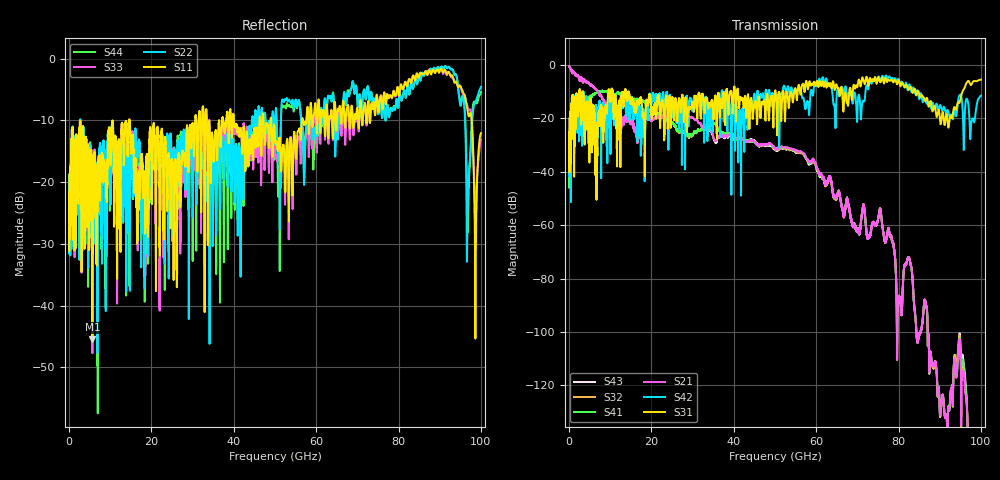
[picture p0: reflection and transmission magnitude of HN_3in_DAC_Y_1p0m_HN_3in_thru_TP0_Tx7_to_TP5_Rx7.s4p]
# GHz S RI R 45
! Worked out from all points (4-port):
!   4000 points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, 25 MHz to 100 GHz, reference 45 ohm
!   strongest paths, dB at 25 MHz, 25.02 GHz, 50.02 GHz, 75.03 GHz, 100 GHz:
!     S31: -39.1, -12.4, -9.7, -4.6, -5.5
!     S42: -38.9, -15.9, -12.9, -4.7, -11.5
!     S21: -0.4, -19.1, -31.1, -57.7, -180.1
!     S41: -45.9, -21.3, -31.3, -57.7, -182.6
!     S32: -45.9, -21.5, -31.2, -57.7, -181.7
!     S43: -0.4, -19.2, -31.5, -57.7, -174.4
!   lowest |S11| = -45.4 dB at 5.675 GHz (marker M1), VSWR 1.01, Z = 44.9 + j0.463 ohm
!   |S11| at or under -10 dB: start of sweep to 10.55 GHz; 14.73 GHz to 30.62 GHz (15.89 GHz wide, 70.1 % of centre); 49.09 GHz to 56.56 GHz (7.47 GHz wide, 14.1 % of centre)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
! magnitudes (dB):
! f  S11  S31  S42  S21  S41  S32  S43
! 25 MHz  -24.2  -39.1  -38.9  -0.4  -45.9  -45.9  -0.4
! 5.675 GHz  -45.4  -20.4  -20.1  -7.8  -11.4  -11.4  -7.8
! 56.58 GHz  -9.9  -7.6  -11.9  -32.7  -32.8  -32.9  -33.1
! 79.9 GHz  -4.9  -6.2  -5.2  -87.4  -87.4  -87.3  -87.3
! 91.67 GHz  -2.5  -18.2  -17.8  -131.2  -131.1  -131.2  -131.1
! 96.9 GHz  -9.0  -6.0  -14.2  -143.2  -139.6  -142.9  -138.3
! 100 GHz  -12.1  -5.5  -11.5  -180.1  -182.6  -181.7  -174.4
